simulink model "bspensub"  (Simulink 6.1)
settings: Solver=ode45  SolverMode=SingleTasking  StartTime=0.0  StopTime=10.0  FixedStep=0.01  RelTol=1e-3

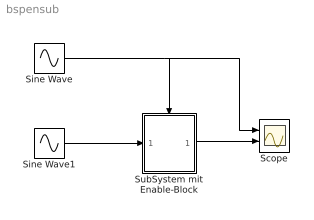
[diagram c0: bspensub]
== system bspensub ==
  Scope : Scope  NumInputPorts=2
  Sine Wave : Sin  SampleTime=0
  Sine Wave1 : Sin  SampleTime=0
  SubSystem mit Enable-Block : Subsystem
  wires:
  SubSystem mit Enable-Block/1(Out1) -> Scope/2
  Sine Wave1/1 -> SubSystem mit Enable-Block/1(In1)
  Sine Wave/1 -> SubSystem mit Enable-Block/Enable, Scope/1

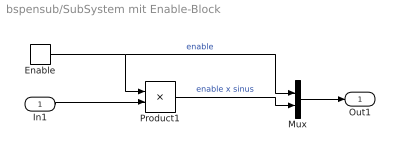
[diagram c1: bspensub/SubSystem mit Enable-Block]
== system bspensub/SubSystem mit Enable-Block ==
  In1 : Inport  Port=1  LatchInput=off
  Enable : EnablePort  ShowOutputPort=on
  Mux : Mux  Inputs=2
  Product1 : Product  Inputs=**
  Out1 : Outport
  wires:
  In1/1 -> Product1/2
  Product1/1 -> Mux/2  "enable x sinus"
  Enable/1 -> Product1/1, Mux/1  "enable"
  Mux/1 -> Out1/1
